(* Logix 5000 AddOnInstructionDefinition export AMCI_SV160E2_Registration_Move_CCW; software revision 20.03 *)

ADD_ON_INSTRUCTION AMCI_SV160E2_Registration_Move_CCW   (* revision 1.0, vendor AMCI, ExecuteEnableInFalse *)
// Revision note:
// 8/2019 Version 0 Initial release of SV160E2 Add On Instructions.
// 3/17/20 Version 1 replaced the generic EDS file with a more complete V1.6 EDS file.
VAR_INPUT
   Status_Word_0 : INT; {required}
   Status_Word_1 : INT; {required}
   Type_0_for_standard_1_for_indexed : BOOL;
   Stopping_Distance : DINT; {required}
   Programmed_Speed : DINT; {required}
   Acceleration : INT; {required}
   Deceleration : INT; {required}
   Minimum_Registration_Move_Distance : DINT; {required}
END_VAR
VAR_IN_OUT
   AMCI_SV160E2_output_data : _000A:SV160E2_9125ACD4:O:0; {required}
END_VAR
VAR_OUTPUT
   EN : BOOL; {visible}
   Registration_Move_CW_Occurring : BOOL; {access Read Only, visible}
   ER : BOOL; {visible}
END_VAR
VAR
   Upper_Result_X_1000 : DINT;
   command_data_block : INT[10];
        [0]   // Command Bits MSW
        [1]   // Command Bits LSW
        [2]   // Upper Target Position
        [3]   // Lower Target Position
        [4]   // Upper Programmed Speed
        [5]   // Lower Programmed Speed
END_VAR

ROUTINE EnableInFalse   (* ladder *)
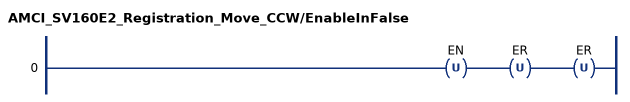
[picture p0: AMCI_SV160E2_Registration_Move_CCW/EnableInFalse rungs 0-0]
   0: OTU(EN)OTU(ER)OTU(ER);
END_ROUTINE

ROUTINE Logic   (* ladder *)
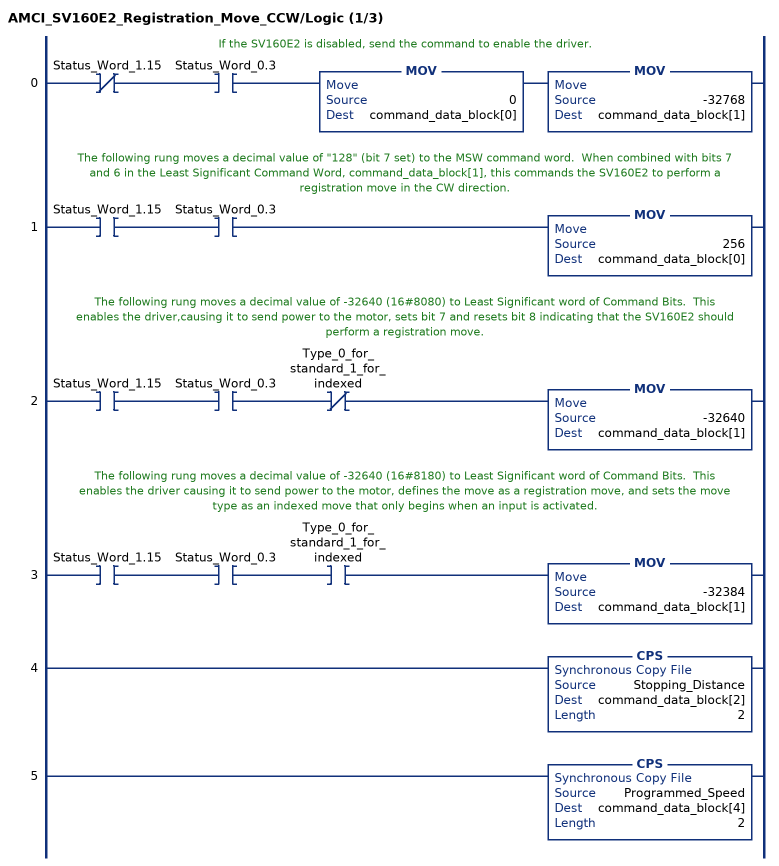
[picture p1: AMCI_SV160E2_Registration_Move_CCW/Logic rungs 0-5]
   // If the SV160E2 is disabled, send the command to enable the driver.
   0: XIO(Status_Word_1.15)XIC(Status_Word_0.3)MOV(0,command_data_block[0])MOV(-32768,command_data_block[1]);
   // The following rung moves a decimal value of "128" (bit 7 set) to the MSW command word.  When combined with bits 7 and 6 in the Least Significant Command Word, command_data_block[1], this commands the SV160E2 to perform a registration move in the CW direction.
   1: XIC(Status_Word_1.15)XIC(Status_Word_0.3)MOV(256,command_data_block[0]);
   // The following rung moves a decimal value of -32640 (16#8080) to Least Significant word of Command Bits.  This enables the driver,causing it to send power to the motor, sets bit 7 and resets bit 8 indicating that the SV160E2 should perform a registration move.
   2: XIC(Status_Word_1.15)XIC(Status_Word_0.3)XIO(Type_0_for_standard_1_for_indexed)MOV(-32640,command_data_block[1]);
   // The following rung moves a decimal value of -32640 (16#8180) to Least Significant word of Command Bits.  This enables the driver causing it to send power to the motor, defines the move as a registration move, and sets the move type as an indexed move that only begins when an input is activated.
   3: XIC(Status_Word_1.15)XIC(Status_Word_0.3)XIC(Type_0_for_standard_1_for_indexed)MOV(-32384,command_data_block[1]);
   4: CPS(Stopping_Distance,command_data_block[2],2);
   5: CPS(Programmed_Speed,command_data_block[4],2);
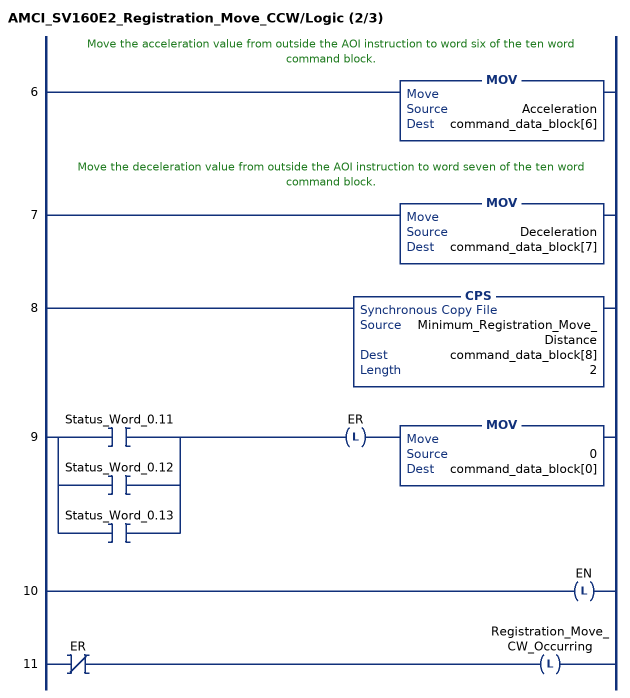
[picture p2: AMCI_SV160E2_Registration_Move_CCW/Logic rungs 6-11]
   // Move the acceleration value from outside the AOI instruction to word six of the ten word command block.
   6: MOV(Acceleration,command_data_block[6]);
   // Move the deceleration value from outside the AOI instruction to word seven of the ten word command block.
   7: MOV(Deceleration,command_data_block[7]);
   8: CPS(Minimum_Registration_Move_Distance,command_data_block[8],2);
   9: [XIC(Status_Word_0.11) ,XIC(Status_Word_0.12) ,XIC(Status_Word_0.13) ]OTL(ER)MOV(0,command_data_block[0]);
   10: OTL(EN);
   11: XIO(ER)OTL(Registration_Move_CW_Occurring);
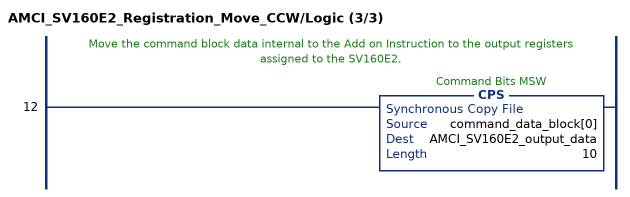
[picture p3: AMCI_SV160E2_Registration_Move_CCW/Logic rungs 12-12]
   // Move the command block data internal to the Add on Instruction to the output registers assigned to the SV160E2.
   12: CPS(command_data_block[0],AMCI_SV160E2_output_data,10);
END_ROUTINE
END_ADD_ON_INSTRUCTION
